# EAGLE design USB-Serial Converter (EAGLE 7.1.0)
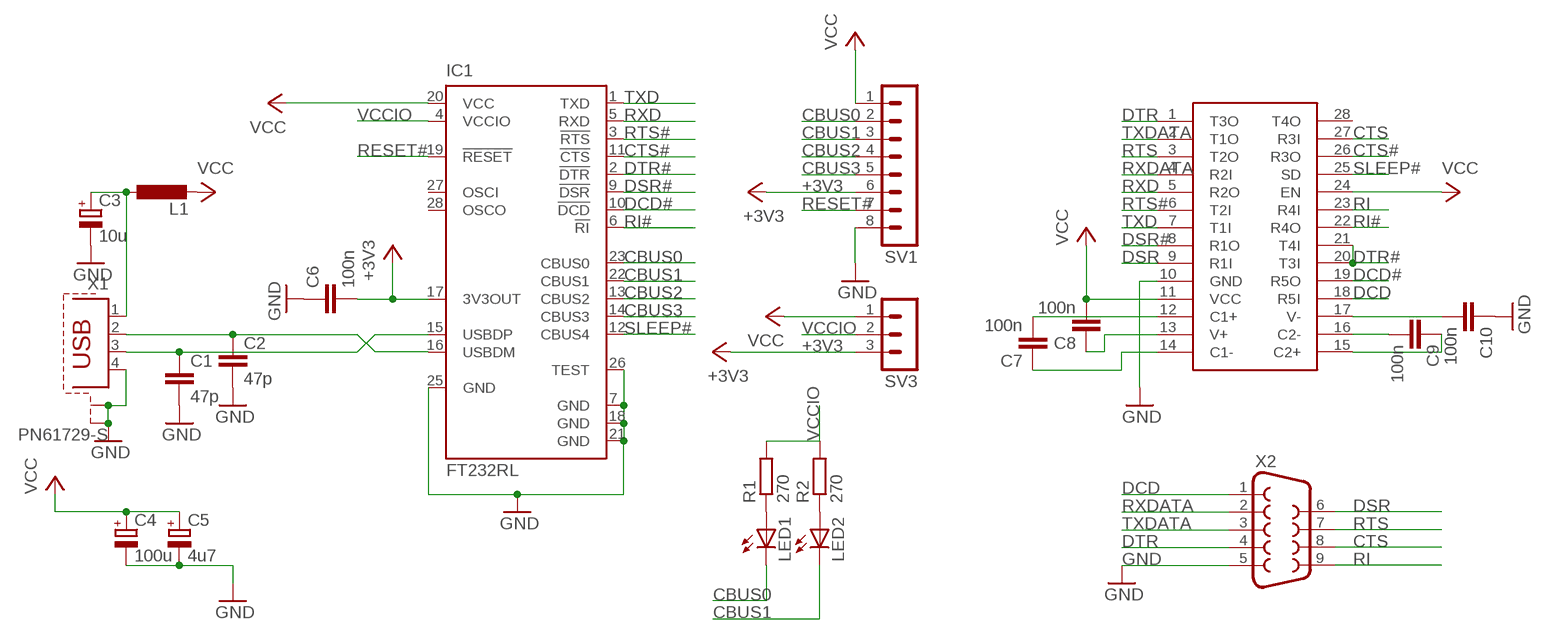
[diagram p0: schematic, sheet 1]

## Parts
C1  47p  C-EUC1206K  [C1206K]
C2  47p  C-EUC1206K  [C1206K]
C3  10u  CPOL-EU153CLV-0505  [153CLV-0505]
C4  100u  CPOL-EU153CLV-0807  [153CLV-0807]
C5  4u7  CPOL-EU153CLV-0505  [153CLV-0505]
C6  100n  C-EUC1206K  [C1206K]
C7  100n  C-EUC1206K  [C1206K]
C8  100n  C-EUC1206K  [C1206K]
C9  100n  C-EUC1206K  [C1206K]
C10  100n  C-EUC1206K  [C1206K]
IC1  FT232RL  [SSOP28]
L1  L-EUL4532P  [L4532P]
LED1  LEDCHIPLED_1206  [CHIPLED_1206]
LED2  LEDCHIPLED_1206  [CHIPLED_1206]
R1  270  R-EU_M1206  [M1206]
R2  270  R-EU_M1206  [M1206]
SV1  MA08-1  [MA08-1]
SV3  MA03-1  [MA03-1]
U$1  SP213EHCA  [SOIC]
X1  PN61729-S  [PN61729-S]
X2  F09HP  [F09HP]

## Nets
+3V3: C6.2 IC1.17(3V3OUT) SV1.6 SV3.3
CBUS0: IC1.23(CBUS0) LED1.C SV1.2
CBUS1: IC1.22(CBUS1) LED2.C SV1.3
CBUS2: IC1.13(CBUS2) SV1.4
CBUS3: IC1.14(CBUS3) SV1.5
CTS: U$1.27(R3I) X2.8
CTS#: IC1.11(!CTS) U$1.26(R3O)
DCD: U$1.18(R5I) X2.1
DCD#: IC1.10(!DCD) U$1.19(R5O)
DSR: U$1.9(R1I) X2.6
DSR#: IC1.9(!DSR) U$1.8(R1O)
DTR: U$1.1(T3O) X2.4
DTR#: IC1.2(!DTR) U$1.20(T3I) U$1.21(T4I)
GND: C1.2 C2.2 C3.- C4.- C5.- C6.1 C10.1 IC1.7(GND) IC1.18(GND) IC1.21(GND) IC1.25(GND) IC1.26(TEST) SV1.8 U$1.10(GND) X1.4 X1.S1 X1.S2 X2.5
N$1: C3.+ L1.1 X1.1
N$2: C1.1 IC1.15(USBDP) X1.3
N$3: C2.1 IC1.16(USBDM) X1.2
N$4: LED1.A R1.1
N$5: LED2.A R2.1
N$14: C7.1 U$1.14(C1-)
N$15: C8.1 U$1.13(V+)
N$16: C7.2 U$1.12(C1+)
N$31: C10.2 U$1.17(V-)
N$32: C9.2 U$1.16(C2-)
N$33: C9.1 U$1.15(C2+)
RESET#: IC1.19(!RESET) SV1.7
RI: U$1.23(R4I) X2.9
RI#: IC1.6(!RI) U$1.22(R4O)
RTS: U$1.3(T2O) X2.7
RTS#: IC1.3(!RTS) U$1.6(T2I)
RXD: IC1.5(RXD) U$1.5(R2O)
RXDATA: U$1.4(R2I) X2.2
SLEEP#: IC1.12(CBUS4) U$1.25(SD)
TXD: IC1.1(TXD) U$1.7(T1I)
TXDATA: U$1.2(T1O) X2.3
VCC: C4.+ C5.+ C8.2 IC1.20(VCC) L1.2 SV1.1 SV3.1 U$1.11(VCC) U$1.24(EN)
VCCIO: IC1.4(VCCIO) R1.2 R2.2 SV3.2
Unconnected: IC1.27(OSCI) IC1.28(OSCO) U$1.28(T4O)

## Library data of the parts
C1 C2 C6-C10 = rcl:C-EU: CAPACITOR, European symbol
C3-C5 = rcl:CPOL-EU: POLARIZED CAPACITOR, European symbol
IC1 = ftdichip:FT232R: Source: http://www.ftdichip.com/Documents/DataSheets/DS_FT232R_v104.pdf; MPN: FT232RL; OC_FARNELL: 1146032; OC_NEWARK: 91K9918
L1 = rcl:L-EU: INDUCTOR, European symbol
LED1 LED2 = led:LED: LED
R1 R2 = rcl:R-EU_: RESISTOR, European symbol
SV1 = con-lstb:MA08-1: PIN HEADER; OC_FARNELL: unknown; OC_NEWARK: unknown
SV3 = con-lstb:MA03-1: PIN HEADER; OC_FARNELL: unknown; OC_NEWARK: unknown
U$1 = sipex:SP213EHCA
X1 = con-berg:PN61729-S: BERG USB connector; OC_FARNELL: unknown; OC_NEWARK: unknown
X2 = con-subd:F09: SUB-D; OC_FARNELL: unknown; OC_NEWARK: unknown

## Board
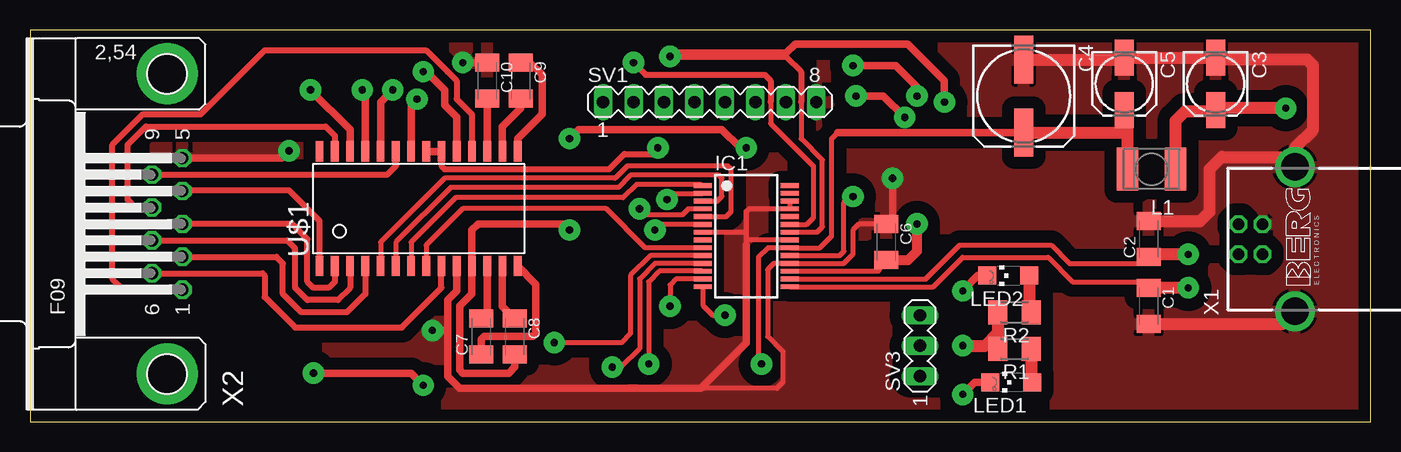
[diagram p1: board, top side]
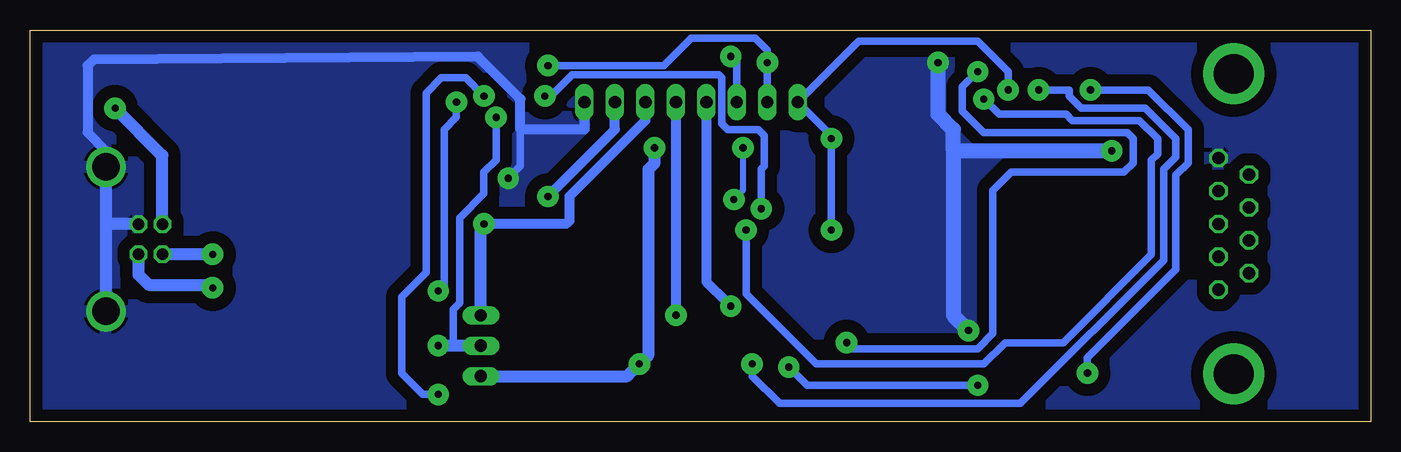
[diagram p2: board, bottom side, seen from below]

Size 111.74 x 32.69 mm. Coordinates in mm from the lower left corner, seen from the top.
Outline: 0,0 111.74,0 111.74,32.69 0,32.69 0,0
Copper layers (1*16): Top 0.035mm / dielectric 1.5mm / Bottom 0.035mm
Design rules "default": minimum track width 10mil, minimum drill 24mil, track to track 8mil, track to pad 8mil, pad to pad 8mil, via to via 8mil, smd to smd 8mil, copper to edge 40mil, drill to drill 8mil, minimum pad ring 10mil, minimum via ring 8mil, stop-mask expansion 4mil, vias tented up to drill 0mil, thermal gap 10mil

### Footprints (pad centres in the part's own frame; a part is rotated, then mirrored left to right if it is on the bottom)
C1206K = smd 1.5 x 2: 1 -1.5,0; 2 1.5,0
153CLV-0505 = smd 3 x 1.6: + 2.2,0; - -2.2,0
153CLV-0807 = smd 4 x 1.6: + 3.05,0; - -3.05,0
SSOP28 = smd 0.4 x 1.5: 1 -4.225,-3.625; 2 -3.575,-3.625; 3 -2.925,-3.625; 4 -2.275,-3.625; 5 -1.625,-3.625; 6 -0.975,-3.625; 7 -0.325,-3.625; 8 0.325,-3.625; 9 0.975,-3.625; 10 1.625,-3.625; 11 2.275,-3.625; 12 2.925,-3.625; 13 3.575,-3.625; 14 4.225,-3.625; 15 4.225,3.625; 16 3.575,3.625; 17 2.925,3.625; 18 2.275,3.625; 19 1.625,3.625; 20 0.975,3.625; 21 0.325,3.625; 22 -0.325,3.625; 23 -0.975,3.625; 24 -1.625,3.625; 25 -2.275,3.625; 26 -2.925,3.625; 27 -3.575,3.625; 28 -4.225,3.625
L4532P = smd 1.8 x 3.6: 1 -2,0; 2 2,0
CHIPLED_1206 = smd 1.5 x 1.5: A 0,-1.75; C 0,1.75
M1206 = smd 1.6 x 2: 1 -1.4,0; 2 1.4,0
MA08-1 = drill 1.016 long: 1 -8.89,0; 2 -6.35,0; 3 -3.81,0; 4 -1.27,0; 5 1.27,0; 6 3.81,0; 7 6.35,0; 8 8.89,0
MA03-1 = drill 1.016 long: 1 -2.54,0; 2 0,0; 3 2.54,0
SOIC = smd 0.65 x 1.7: 1 -7.62,-4.78; 2 -6.35,-4.78; 3 -5.08,-4.78; 4 -3.81,-4.78; 5 -2.54,-4.78; 6 -1.27,-4.78; 7 0,-4.78; 8 1.27,-4.78; 9 2.54,-4.78; 10 3.81,-4.78; 11 5.08,-4.78; 12 6.35,-4.78; 13 7.62,-4.78; 14 8.89,-4.78; 15 8.89,4.78; 16 7.62,4.78; 17 6.35,4.78; 18 5.08,4.78; 19 3.81,4.78; 20 2.54,4.78; 21 1.27,4.78; 22 0,4.78; 23 -1.27,4.78; 24 -2.54,4.78; 25 -3.81,4.78; 26 -5.08,4.78; 27 -6.35,4.78; 28 -7.62,4.78
PN61729-S = drill 0.95 octagon: 1 1.25,4.71; 2 -1.25,4.71; 3 -1.25,2.71; 4 1.25,2.71 | drill 2.3 pad 2.9: S1 -6.02,0; S2 6.02,0
F09HP = drill 1.016 octagon: 1 -5.486,-1.27; 2 -2.743,-1.27; 3 0,-1.27; 4 2.743,-1.27; 5 5.486,-1.27; 6 -4.115,1.27; 7 -1.372,1.27; 8 1.372,1.27; 9 4.115,1.27 | drill 3.302 pad 5.08: G1 -12.522,0; G2 12.522,0

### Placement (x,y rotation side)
C1  93.22,9.65 270 top
C2  93.22,15.24 90 top
C3  98.81,28.19 270 top
C4  82.8,27.18 270 top
C5  91.19,28.19 270 top
C6  71.37,14.99 270 top
C7  37.59,7.11 90 top
C8  40.39,7.11 270 top
C9  40.89,28.45 270 top
C10  38.1,28.45 270 top
IC1  59.69,15.49 270 top
L1  93.47,21.08 180 top
LED1  81.79,3.3 90 top
LED2  81.53,12.19 90 top
R1  82.04,6.1 180 top
R2  82.04,9.14 180 top
SV1  56.64,26.67 0 top
SV3  74.17,6.35 90 top
U$1  31.75,17.78 0 top
X1  105.41,15.24 90 top
X2  11.43,16.51 90 top

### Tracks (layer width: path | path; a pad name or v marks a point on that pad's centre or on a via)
+3V3  (via drill 0.6 pad 1.78)
  Top 0.406: IC1.17 70.71,12.57 C6.2
  Top 0.813: v73.91,16.51 73.91,14.22 73.15,13.46 71.4,13.46 C6.2
  Bottom 0.813: SV1.6 60.45,25.15 66.8,18.8 66.8,16.76 67.06,16.51 v73.91,16.51
  Bottom 1.016: SV3.3 74.17,16.26 v73.91,16.51
CBUS0  (via drill 0.6 pad 1.78)
  Top 0.406: 61.72,26.67 61.72,24.89 65.28,21.34 65.28,17.02 64.73,16.47 IC1.23
  Top 0.508: v50.29,29.97 51.31,28.96 61.21,28.96 61.72,28.45 61.72,26.67
  Top 0.61: LED1.C 78.74,3.3 v77.72,2.29 | v73.91,27.18 73.91,27.94 72.14,29.72 v68.58,29.72
  Bottom 0.61: SV1.2 v50.29,29.97 50.29,30.99 51.31,32 56.64,32 58.93,29.72 v68.58,29.72 | v77.72,2.29 78.99,2.29 80.77,4.06 80.77,10.41 78.74,12.45 78.74,27.43 77.47,28.7 75.44,28.7 v73.91,27.18
CBUS1  (via drill 0.6 pad 1.78)
  Top 0.406: 64.26,26.67 64.26,23.62 66.04,21.84 66.04,16.26 65.6,15.82 IC1.22
  Top 0.508: v53.34,30.48 62.99,30.48 64.26,29.21 64.26,26.67
  Top 0.61: LED2.C 78.99,12.19 v77.72,10.92 | v76.2,26.67 76.2,28.45 73.15,31.5 63.75,31.5 62.99,30.73 53.59,30.73 v53.34,30.48
  Bottom 0.61: SV1.3 52.83,29.97 v53.34,30.48 | v77.72,10.92 77.22,11.43 77.22,24.38 76.2,25.4 v76.2,26.67
CBUS2  (via drill 0.6 pad 1.78)
  Top 0.406: IC1.13 53.83,11.92 53.34,11.43 v53.34,9.65
  Bottom 0.813: SV1.4 55.37,11.68 53.72,10.03 v53.34,9.65
CBUS3  (via drill 0.6 pad 1.78)
  Top 0.406: IC1.14 56.06,9.72 56.9,8.89 v57.91,8.89
  Bottom 0.813: SV1.5 57.91,9.65 v57.91,8.89
CTS
  Top 0.508: X2.8 8.79,17.88 8.13,18.54 8.13,23.11 9.65,24.64 24.64,24.64 25.4,23.88 U$1.27
CTS#  (via drill 0.6 pad 1.78)
  Top 0.406: v48.51,4.57 49.28,4.57 50.8,6.1 50.8,11.94 52.08,13.22 IC1.11
  Top 0.61: U$1.26 26.67,24.38 v23.37,27.69 | v23.62,4.06 31.75,4.06 v32.77,3.05
  Bottom 0.61: v23.37,27.69 23.11,27.69 18.54,27.69 15.24,24.38 15.24,21.59 16.26,20.57 16.26,12.7 23.62,5.33 v23.62,4.06 | v32.77,3.05 46.99,3.05 v48.51,4.57
DCD
  Top 0.508: X2.1 7.77,11.02 6.86,11.94 6.86,23.11 9.4,25.65 14.22,25.65 19.56,30.99 30.48,30.99 33.02,30.99 34.8,29.21 35.56,28.45 35.56,26.92 36.83,25.65 U$1.18
DCD#  (via drill 0.6 pad 1.78)
  Top 0.406: IC1.10 51.72,13.87 50.04,12.19 50.04,7.37 49.28,6.6 v43.69,6.6
  Top 0.61: v32.77,29.21 33.02,29.21 34.54,27.69 34.54,26.42 35.56,25.4 U$1.19
  Bottom 0.61: v43.69,6.6 43.18,6.1 32.77,6.1 31.5,7.37 31.5,19.3 29.97,20.83 20.57,20.83 19.81,21.59 19.81,23.62 20.32,24.13 32.26,24.13 34.04,25.91 34.04,27.94 v32.77,29.21
DSR
  Top 0.508: X2.6 19.36,12.39 19.56,12.19 19.56,10.41 22.1,7.87 30.99,7.87 34.29,11.18 U$1.9
DSR#
  Top 0.406: IC1.9 51.27,14.52 48.01,17.78 36.07,17.78 33.02,14.73 U$1.8
DTR
  Top 0.508: U$1.1 24.13,16.76 21.59,19.3 12.75,19.3 X2.4
DTR#  (via drill 0.6 pad 1.78)
  Top 0.406: v53.09,18.54 53.59,19.05 56.05,19.05 IC1.2
  Top 0.508: U$1.20 34.29,21.34 34.54,21.08 48.26,21.08 49.53,22.35 51.82,22.35 v52.32,22.86
  Top 0.61: U$1.21 U$1.20
  Bottom 0.508: v52.32,22.86 52.32,19.3 v53.09,18.54
GND  (via drill 0.6 pad 1.78)
  Top 0.406: IC1.7 59.62,15.82 | 59.93,17.77 IC1.25 IC1.26 | IC1.21 59.76,15.17 | C6.1 69.06,16.49 68.58,16 68.58,13.97 67.83,13.22 IC1.18 61.99,13.22 61.47,12.7 61.47,7.11 62.74,5.84 62.74,3.3 62.23,2.79 56.13,2.79 56.01,2.92
  Top 0.457: 59.69,14.22 59.69,14.73 59.69,15.24 | 59.69,15.24 59.69,15.75 | 59.69,15.75 59.69,17.53 59.93,17.77 | 59.76,15.17 59.69,15.24 | 59.62,15.82 59.69,15.75
  Top 0.61: v71.88,20.32 71.88,16.99 C6.1 | U$1.10 35.56,10.92 34.8,10.16 34.8,7.62 | 34.8,7.62 34.8,3.81 35.81,2.79 55.88,2.79 56.01,2.92 59.69,6.6 59.69,14.73 | X2.5 20.98,22 v21.59,22.61 | v33.53,7.62 34.8,7.62 | C10.1 36.09,29.95 v36.07,29.97
  Top 1.016: C4.- 91.02,30.23 C5.- C3.- 98.97,30.23 106.43,30.23 106.93,29.72 106.93,24.38 105.41,22.86 105.41,22.1 | X1.S2 105.41,22.1 | C2.2 97.51,16.74 98.3,17.53 98.3,21.08 99.31,22.1 105.41,22.1 | C1.2 104.34,8.15 X1.S1
  Bottom 0.61: 70.87,24.38 70.87,21.34 v71.88,20.32
  Bottom 0.813: SV1.8 65.53,24.38 70.87,24.38 70.87,26.92 74.42,30.48 106.43,30.23 106.93,29.72 106.93,24.13 105.41,22.61 X1.S2
  Bottom 1.016: X1.S2 105.41,16.76 | 105.41,16.76 X1.S1 | X1.4 105.14,16.49 105.41,16.76
  Bottom 1.27: v21.59,22.61 34.8,22.61 | 34.8,22.61 34.8,24.38 36.07,25.65 v36.07,29.97 | 34.8,22.61 34.8,8.89 v33.53,7.62
  pour Top (isolate 1.016): -1.02,34.54 114.81,34.54 114.81,-2.79 -3.05,-2.79 -3.05,34.54
  pour Bottom (isolate 1.016): -3.3,34.8 112.52,34.8 112.52,-2.54 -5.33,-2.54 -5.33,34.8
N$1  (via drill 0.6 pad 1.78)
  Top 1.016: v104.65,26.16 98.97,26.16 C3.+ 98.72,25.91 96.27,25.91 95.47,25.11 L1.1
  Bottom 1.016: X1.1 100.7,22.21 v104.65,26.16
N$2  (via drill 0.6 pad 1.78)
  Top 0.406: IC1.15 75.28,11.27 77.72,13.72 84.84,13.72 86.87,11.68 93.47,11.68 C1.1
  Top 1.016: v96.52,11.18 93.24,11.18 C1.1
  Bottom 1.016: X1.3 102.7,12.28 101.85,11.43 96.77,11.43 v96.52,11.18
N$3  (via drill 0.6 pad 1.78)
  Top 0.406: IC1.16 74.66,11.92 77.47,14.73 85.09,14.73 86.61,13.21 92.96,13.21 C2.1
  Top 1.016: v96.52,13.97 93.45,13.97 C2.1
  Bottom 1.016: X1.2 96.54,13.99 v96.52,13.97
N$4
  Top 1.016: R1.1 83.44,3.4 LED1.A
N$5
  Top 1.016: LED2.A 83.28,9.3 R2.1
N$14
  Top 0.61: C7.1 37.59,6.86 37.85,7.11 41.91,7.11 42.16,7.37 42.16,11.48 U$1.14
N$15
  Top 0.61: U$1.13 39.37,9.63 C8.1
N$16
  Top 0.61: U$1.12 38.1,9.12 C7.2
N$31
  Top 0.61: U$1.17 C10.2
N$32
  Top 0.61: U$1.16 39.37,24.64 40.89,26.16 C9.2
N$33
  Top 0.61: U$1.15 40.64,23.62 42.67,25.65 42.67,28.96 41.66,29.97 40.92,29.97 C9.1
RESET#  (via drill 0.6 pad 1.78)
  Top 0.406: IC1.19 67.46,13.87 67.82,14.22 67.82,18.29 68.33,18.8 v68.58,18.8
  Bottom 0.813: v68.58,18.8 62.99,24.38 SV1.7
RI
  Top 0.508: X2.9 29.77,20.62 30.48,21.34 U$1.23
RI#  (via drill 0.6 pad 1.78)
  Top 0.406: IC1.6 52.37,16.47 v52.07,16
  Top 0.61: U$1.22 31.75,26.42 v32.26,26.92
  Bottom 0.61: v32.26,26.92 30.99,25.65 25.4,25.65 24.89,25.15 19.3,25.15 17.78,23.62 17.78,22.35 18.29,21.84 18.29,13.97 25.65,6.6 30.48,6.6 32.26,4.83 46.23,4.83 52.07,10.67 v52.07,16
RTS
  Top 0.508: U$1.3 26.67,11.18 25.65,10.16 23.11,10.16 22.1,11.18 22.1,14.48 21.44,15.14 X2.7
RTS#
  Top 0.406: IC1.3 57.28,18.42 57.66,18.8 57.66,20.32 57.4,20.57 50.04,20.57 49.02,19.56 35.05,19.56 30.48,14.99 U$1.6
RXD
  Top 0.406: IC1.5 58.01,17.12 58.42,17.53 58.42,21.08 58.17,21.34 49.78,21.34 48.77,20.32 34.54,20.32 29.21,14.99 U$1.5
RXDATA
  Top 0.508: U$1.4 27.94,10.67 26.42,9.14 22.61,9.14 21.08,10.67 21.08,13.21 20.52,13.77 X2.2
SLEEP#  (via drill 0.6 pad 1.78)
  Top 0.406: IC1.12 52.45,12.57 51.56,11.68 v51.56,4.83
  Top 0.61: v27.69,27.69 27.94,27.43 U$1.25
  Bottom 0.61: v51.56,4.83 51.56,3.81 49.28,1.52 29.21,1.52 17.27,13.46 17.27,21.08 16.26,22.1 16.26,23.62 18.8,26.16 24.13,26.16 25.15,27.18 25.15,27.69 v27.69,27.69
TXD
  Top 0.406: IC1.1 55.88,19.81 50.55,19.81 49.44,18.7 35.47,18.7 31.75,14.99 U$1.7
TXDATA
  Top 0.508: U$1.2 25.4,11.68 24.89,11.18 23.62,11.18 23.11,11.68 23.11,15.24 21.84,16.51 X2.3
VCC  (via drill 0.6 pad 1.78)
  Top 0.406: 67.31,24.13 66.8,23.62 66.8,15.49 65.83,14.52 IC1.20 61.51,14.52 60.71,13.72 60.71,5.08 v60.96,4.83
  Top 0.61: 67.31,24.13 83.31,24.13 | C8.2 40.39,4.57 39.88,4.06 36.07,4.06 35.81,4.32 35.81,9.65 36.83,10.67 U$1.11 36.83,16 37.34,16.51 44.45,16.51 v44.96,16 | U$1.24 29.21,26.67 v30.23,27.69 | v59.69,22.86 59.18,22.86 57.66,24.38 45.72,24.38 v44.96,23.62
  Top 1.016: L1.2 91.47,24.13 | 91.47,24.13 91.47,25.71 C5.+ | C4.+ 83.31,24.13 91.47,24.13
  Bottom 0.61: v44.96,16 v44.96,23.62 44.96,23.88 SV1.1 42.67,31.75 32.77,31.75 30.23,29.21 v30.23,27.69
  Bottom 1.016: SV3.1 61.98,3.81 61.59,4.19 v60.96,4.83 60.2,5.59 60.2,21.08 59.69,21.59 v59.69,22.86
VCCIO  (via drill 0.6 pad 1.78)
  Top 0.406: IC1.4 54.85,17.77 54.36,17.27 51.31,17.27 v50.8,17.78
  Top 0.61: v68.83,27.18 71.12,27.18 v72.9,25.4
  Top 1.016: R2.2 80.64,7.37 | 80.64,7.37 R1.2 | v77.72,6.35 79.63,6.35 80.64,7.37
  Bottom 0.61: v50.8,17.78 50.8,21.08 50.55,21.34 50.55,23.88 51.05,24.38 53.59,24.38 54.1,24.89 54.1,28.7 54.36,28.96 66.55,28.96 68.33,27.18 v68.83,27.18 | v72.9,25.4 72.9,21.84 73.91,20.83 73.91,19.05 75.95,17.02 75.95,9.91 76.45,9.4 76.45,6.35
  Bottom 1.016: SV3.2 76.45,6.35 v77.72,6.35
